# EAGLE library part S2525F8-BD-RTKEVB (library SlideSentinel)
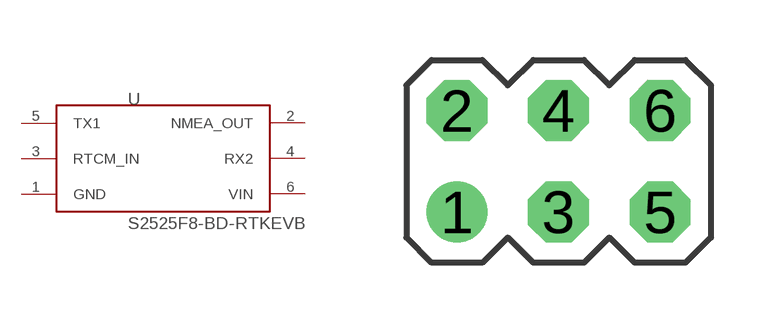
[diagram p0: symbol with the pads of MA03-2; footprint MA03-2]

Designator prefix -

## S2525F8-BD-RTKEVB  [MA03-2]
1  GND
2  NMEA_OUT
3  RTCM_IN
4  RX2
5  TX1
6  VIN

## Footprint MA03-2 (pad centres in mm)
PIN HEADER
drill 1.016: 1 -2.54,-1.27
drill 1.016 octagon: 2 -2.54,1.27; 3 0,-1.27; 4 0,1.27; 5 2.54,-1.27; 6 2.54,1.27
